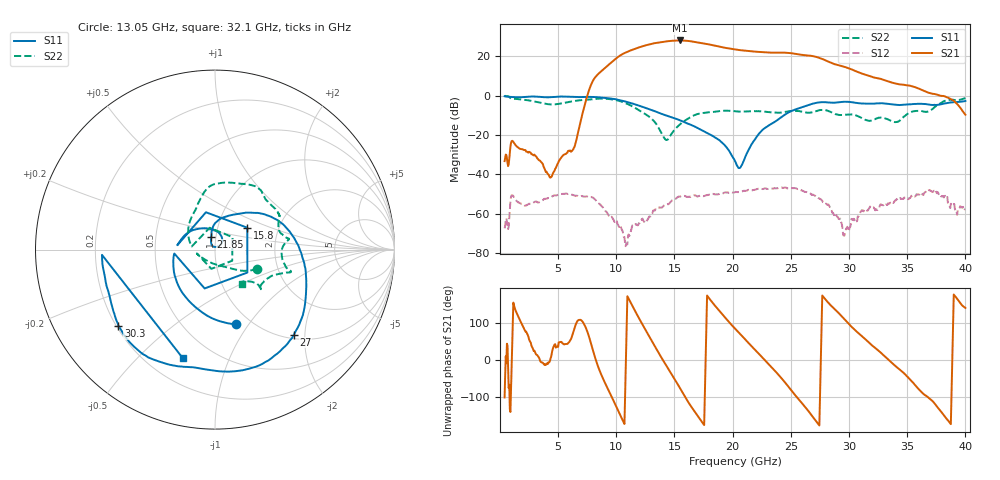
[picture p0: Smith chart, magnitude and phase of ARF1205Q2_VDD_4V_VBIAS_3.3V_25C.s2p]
!Bias:VDD=4.0V, VBIAS=3.3V
# GHz S DB R 50.0
!freq dBS11 angS11 dBS21 angS21 dBS12 angS12 dBS22 angS22
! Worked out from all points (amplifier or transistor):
!   793 points, 400 MHz to 40 GHz, reference 50 ohm
!   highest |S21| = 28.2 dB at 15.5 GHz (marker M1)
!   |S21| within 3 dB of that: 12.23 GHz to 18.73 GHz (6.5 GHz wide, 42 % of centre)
!   unconditionally stable (mu >= 1): 416.1 MHz to end of sweep
!   at 7 GHz: K = 34.36, MAG = 1.5 dB, |S12| = -51.0 dB
!   at 20.2 GHz: K = 7.80, MAG = 24.4 dB, |S12| = -49.0 dB
!   at 40 GHz: K = 119.98, MAG = 0.2 dB, |S12| = -57.7 dB
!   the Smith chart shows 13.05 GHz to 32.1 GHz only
!   S11 on the Smith chart (normalised r, x): 13.05 GHz: 0.85, -0.87; 15.8 GHz: 1.39, +0.36; 21.85 GHz: 0.95, +0.13; 27 GHz: 1.08, -1.76; 30.3 GHz: 0.21, -0.33; 32.1 GHz: 0.34, -0.69
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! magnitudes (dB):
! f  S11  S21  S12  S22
! 400 MHz  -0.2  -33.2  -67.4  0.0
! 1.1 GHz  -0.7  -23.0  -50.7  -1.6
! 4.4 GHz  -0.7  -41.3  -51.6  -4.4
! 6.3 GHz  -0.6  -27.2  -50.5  -2.7
! 7 GHz  -0.6  -11.3  -51.0  -2.2
! 8.1 GHz  -0.6  8.7  -52.4  -1.6
! 10.8 GHz  -2.9  22.0  -76.5  -3.7
! 13.05 GHz  -7.3  26.5  -60.1  -11.7
! 13.6 GHz  -8.5  27.1  -57.0  -15.9
! 14.35 GHz  -10.1  27.7  -55.2  -22.4
! 15.5 GHz  -12.5  28.2  -51.3  -14.4
! 15.8 GHz  -13.3  28.1  -50.9  -13.0
! 20.2 GHz  -33.2  23.6  -49.0  -7.8
! 21.85 GHz  -22.7  22.5  -47.9  -7.8
! 26.8 GHz  -4.1  20.3  -50.5  -8.4
! 27 GHz  -3.8  20.1  -50.6  -8.1
! 29.6 GHz  -3.0  14.8  -71.1  -9.7
! 30.3 GHz  -3.3  13.3  -63.0  -9.5
! 32.1 GHz  -4.0  9.4  -56.7  -12.3
! 33.4 GHz  -4.1  7.3  -55.0  -12.1
! 36.95 GHz  -4.5  1.4  -48.0  -7.6
! 40 GHz  -2.6  -9.6  -57.7  -1.1
